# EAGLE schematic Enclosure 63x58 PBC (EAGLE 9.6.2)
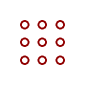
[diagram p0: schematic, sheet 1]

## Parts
U$1  PROTO-20X18-C  [PROTO-20X18-C]

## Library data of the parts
U$1 = digitalconcepts:PROTO-20X18-C: 20 x 18 Prototyping board, with cut-outs, to fit a 63 x 58 enclosure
